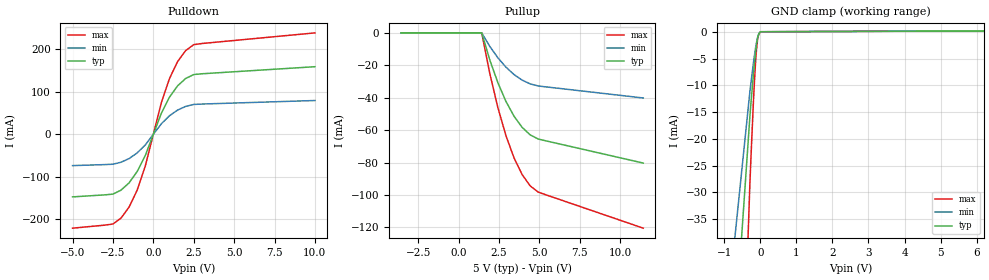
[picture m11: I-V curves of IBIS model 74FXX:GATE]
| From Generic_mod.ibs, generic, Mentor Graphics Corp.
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[Model]   74FXX:GATE
Model_type   I/O
Polarity   Non-Inverting
Vinl  =   0.800V
Vinh  =   2.000V
Vmeas =   1.500V
Cref  =   0.000F
Rref  =   1.000MOhm
Vref  =   0.000V
|   typ   min   max
C_comp   5.000pF   2.500pF   7.500pF
[Voltage Range]   5.000V   4.500V   5.500V
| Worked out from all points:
|   slope of the pulldown table from 0 to 0.75 V, typ, clamps not added: 10.9 ohm
|   GND clamp passes 1 mA (typ) near -0.07 V on its own axis
[Pulldown]
| Voltage   I(typ)   I(min)   I(max)
-5V       -147.2mA   -73.58mA   -220.7mA
-2.5V     -140.6mA   -70.3mA    -210.9mA
-2V       -131.3mA   -65.67mA   -197mA
-1.5V     -114.1mA   -57.04mA   -171.1mA
-1V       -87.45mA   -43.73mA   -131.2mA
-500mV    -50mA      -25mA      -75mA
500mV     50mA       25mA       75mA
1V        87.45mA    43.73mA    131.2mA
1.5V      114.1mA    57.04mA    171.1mA
2V        131.3mA    65.67mA    197mA
3V        142.4mA    71.21mA    213.6mA
10V       159.1mA    79.54mA    238.6mA
[Pullup]
| Voltage   I(typ)   I(min)   I(max)
-3.577V   0A         0A         0A
1.423V    0A         0A         0A
1.923V    -16.67mA   -8.333mA   -25mA
2.423V    -30.7mA    -15.35mA   -46.05mA
2.923V    -42.23mA   -21.12mA   -63.35mA
3.423V    -51.38mA   -25.69mA   -77.06mA
3.923V    -58.23mA   -29.11mA   -87.34mA
4.423V    -62.89mA   -31.45mA   -94.33mA
4.923V    -65.46mA   -32.73mA   -98.19mA
11.42V    -80.28mA   -40.14mA   -120.4mA
[GND Clamp]
| Voltage   I(typ)   I(min)   I(max)
-5V       -477.1mA   -318.8mA   -950.4mA
-292.8mV  -15.86mA   -11.21mA   -28.48mA
-261mV    -13.19mA   -9.409mA   -23.24mA
-194.9mV  -7.964mA   -5.866mA   -13.17mA
-163.1mV  -5.696mA   -4.304mA   -8.933mA
-132mV    -3.732mA   -2.924mA   -5.434mA
-112.1mV  -2.653mA   -2.144mA   -3.63mA
-100.2mV  -2.09mA    -1.726mA   -2.744mA
-71.08mV  -1.017mA   -891.7uA   -1.201mA
-42.9mV   -392uA     -364uA     -426.5uA
0V        0A         0A         0A
10V       128uA      128uA      128uA
[Ramp]
|   typ   min   max
dV/dt_r   1.255V/1.500ns   0.731V/2.700ns   1.675V/1.100ns
dV/dt_f   2.443V/1.080ns   1.750V/1.944ns   2.883V/792.000ps
R_load =  50.000Ohm
|------------------- End of 74FXX:GATE ----------------------------------------
